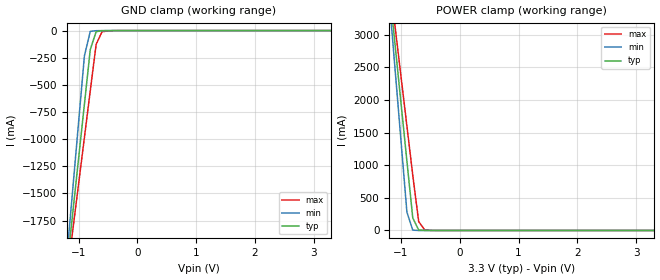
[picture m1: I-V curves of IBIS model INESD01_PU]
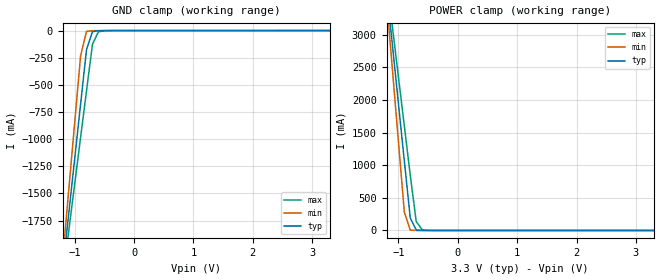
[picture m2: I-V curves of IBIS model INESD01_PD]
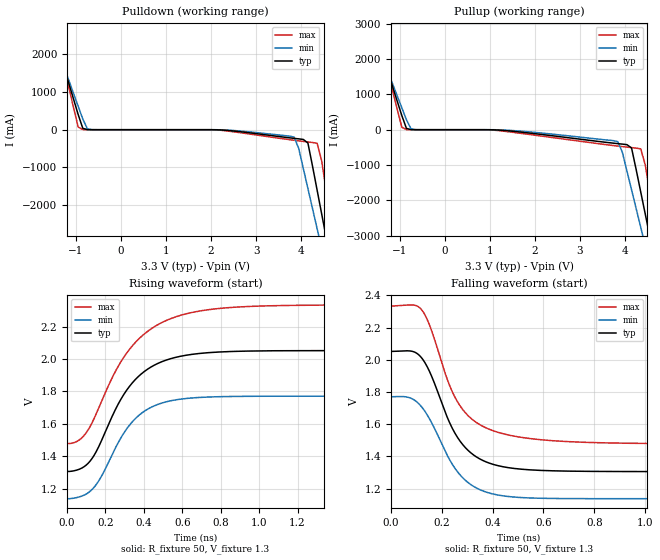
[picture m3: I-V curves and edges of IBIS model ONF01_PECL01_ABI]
|   This file is an IBIS representation of the   |
|   Integrated Devices Technology, Inc.   |
|   ICS84321   |
|   XTAL to 3.3V Differential LVPECL Frequency Synthesizer   |
[IBIS Ver]   4.1
[File name]   84321_3v3.ibs
[File Rev]   1.0
[Date]   31 Dec 2008 | Last modified
|   15 Apr 2003 | Generated
[Source]   Originated at Integrated Devices Technology, Inc.
[Disclaimer]
IDT hereby grants the user of this IBIS model a non-exclusive,
nontransferable license to use this IBIS model under the following terms.
Before using this IBIS model, the user should read this license.
If the user does not accept these terms,  the IBIS model should be
returned to IDT within 30 days.
   The user is granted this license only to use the IBIS model and
is not granted rights to sell, load, rent, lease or license the IBIS
model in whole or in part, or in modified form to anyone other than
user. User may modify the IBIS model to suit its specific
applications but rights to derivative works and such modifications
shall belong to IDT.
   This IBIS model is provided on an "AS IS" basis and IDT makes
absolutely no warranty with respect to the information contained
herein. IDT DISCLAIMS AND CUSTOMER WAIVES ALL WARRANTIES, EXPRESS
OR IMPLIED, INCLUDING WARRANTIES OF MERCHANTABILITY OR FITNESS FOR
A PARTICULAR PURPOSE. The entire risk as to quality and performance
is with the Customer. ACCORDINGLY, IN NO EVENT SHALL THE COMPANY BE
LIABLE FOR ANY DAMAGES, WHETHER IN CONTRACT OR TORT,INCLUDING ANY
LOST PROFITS OR OTHER INCIDENTAL, CONSEQUENTIAL, EXEMPLARY, OR
PUNITIVE DAMAGES ARISING OUT OF THE USE OR APPLICATION OF THE IBIS
model provided in this package. Further, IDT reserves the right to
make changes without notice to any product herein to improve
reliability, function, or design. IDT does not convey any license
under patent rights or any other intellectual property rights,
including those of third parties.
   IDT is not obligated to provide maintenance or support
for the licensed IBIS model.
[Copyright]   Copyright 2003 by Integrated Devices Technology, Inc.
[Component]   ICS84321
[Manufacturer] Integrated Devices Technology, Inc.
[Package]
|LQFP32
|lead+wire  typ   min   max
R_pkg   220.4m   212.5m   238m
L_pkg   1.841n   1.708n   1.974n
C_pkg   0.316p   0.2907p   0.33p
[Pin]   signal_name   model_name   R_pin   L_pin   C_pin
1   M5   INESD01_PU   238m   1.974n   0.330p
2   M6   INESD01_PD   225m   1.841n   0.311p
3   M7   INESD01_PD   218m   1.7745n   0.301p
4   M8   INESD01_PU   213m   1.708n   0.291p
5   NO   INESD01_PU   213m   1.708n   0.291p
6   N1   INESD01_PU   218m   1.7745n   0.301p
7   NC   NC   225m   1.841n   0.311p
8   VEE   GND   238m   1.974n   0.330p
9   TEST   NC   238m   1.974n   0.330p
10   VCC   POWER   225m   1.841n   0.311p
11   FOUT1   ONF01_PECL01_ABI   218m   1.7745n   0.301p
12   nFOUT1   ONF01_PECL01_ABI   213m   1.708n   0.291p
13   VCCO   POWER   213m   1.708n   0.291p
14   FOUT0   ONF01_PECL01_ABI   218m   1.7745n   0.301p
15   nFOUT0   ONF01_PECL01_ABI   225m   1.841n   0.311p
16   VEE   GND   238m   1.974n   0.330p
17   MR   INESD01_PD   238m   1.974n   0.330p
18   S_CLOCK   INESD01_PD   225m   1.841n   0.311p
19   S_DATA   INESD01_PD   218m   1.7745n   0.301p
20   S_LOAD   INESD01_PD   213m   1.708n   0.291p
21   VCCA   POWER   213m   1.708n   0.291p
22   XTAL_SEL   INESD01_PU   218m   1.7745n   0.301p
23   TEST_CLK   INESD01_PD   225m   1.841n   0.311p
24   XTAL_OUT   NC   238m   1.974n   0.330p
25   XTAL_IN   NC   238m   1.974n   0.330p
26   nP_LOAD   INESD01_PD   225m   1.841n   0.311p
27   VCO_SEL   INESD01_PU   218m   1.7745n   0.301p
28   M0   INESD01_PD   213m   1.708n   0.291p
29   M1   INESD01_PD   213m   1.708n   0.291p
30   M2   INESD01_PD   218m   1.7745n   0.301p
31   M3   INESD01_PD   225m   1.841n   0.311p
32   M4   INESD01_PD   238m   1.974n   0.330p
[Diff Pin]  inv_pin  vdiff tdelay_typ tdelay_min  tdelay_max
11   12   NA   0  0  0
14   15   NA   0  0  0
| Models and submodels in the file (3): INESD01_PU (Input), INESD01_PD (Input), ONF01_PECL01_ABI (Output_ECL)
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[Model]   INESD01_PU
Model_type   Input
Polarity   Non-Inverting
Vinl = 0.8V
Vinh = 2.0V
|   typ   min   max
C_comp   2pF   1.5pF   2.5pF
|   typ   min   max
[Voltage range]  3.3V   3.15V   3.45V
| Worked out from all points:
|   GND clamp passes 1 mA (typ) near -0.55 V on its own axis
|   POWER clamp passes 1 mA (typ) near -0.61 V on its own axis
[GND_clamp]
|Voltage   I(typ)   I(min)   I(max)
-3.3V     -12.83A    -15.14A    -11.37A
-1.2V     -2.195A    -2.092A    -2.281A
-1.1V     -1.689A    -1.472A    -1.849A
-900mV    -678.5mA   -232.7mA   -984.8mA
-800mV    -174mA     -7.237mA   -553.3mA
-700mV    -9.767mA   -1.114mA   -126.1mA
-600mV    -1.7mA     -240.1uA   -11.15mA
-300mV    -81.66uA   -67.79uA   -163.4uA
3.3V      1.866nA    1.113pA    239.1nA
[POWER_clamp]
|Voltage   I(typ)   I(min)   I(max)
-3.3V     22.38A     26.45A     19.82A
-1.2V     3.723A     3.545A     3.874A
-1.1V     2.836A     2.457A     3.116A
-1V       1.949A     1.369A     2.358A
-900mV    1.063A     281mA      1.601A
-800mV    191.5mA    5.012mA    843.9mA
-700mV    8.032mA    142.2uA    138.3mA
-600mV    607uA      17.63uA    10.62mA
-400mV    16.32uA    7.545uA    335.9uA
3.3V      -71.13uA   -62.11uA   -78.26uA
[Model]   INESD01_PD
Model_type   Input
Polarity   Non-Inverting
Vinl = 0.80V
Vinh = 2.0V
|   typ   min   max
C_comp   2pF   1.5pF   2.5pF
|   typ   min   max
[Voltage range]  3.3V   3.15V   3.45V
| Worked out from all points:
|   GND clamp passes 1 mA (typ) near -0.55 V on its own axis
|   POWER clamp passes 1 mA (typ) near -0.60 V on its own axis
[GND_clamp]
|Voltage I(typ)   I(min)   I(max)
-3.3V     -12.83A    -15.14A    -11.37A
-1.2V     -2.195A    -2.092A    -2.281A
-1.1V     -1.689A    -1.472A    -1.849A
-900mV    -678.5mA   -232.6mA   -984.8mA
-800mV    -173.9mA   -7.175mA   -553.2mA
-700mV    -9.696mA   -1.052mA   -126mA
-600mV    -1.629mA   -178uA     -11.07mA
-300mV    -10.53uA   -5.678uA   -86.08uA
3.3V      71.13uA    62.11uA    77.58uA
[POWER_clamp]
|Voltage   I(typ)   I(min)   I(max)
-3.3V     22.38A     26.45A     19.82A
-1.2V     3.723A     3.545A     3.874A
-1.1V     2.836A     2.457A     3.116A
-1V       1.949A     1.369A     2.358A
-900mV    1.063A     281.1mA    1.601A
-800mV    191.6mA    5.074mA    844mA
-700mV    8.104mA    204.3uA    138.4mA
-600mV    678.1uA    79.74uA    10.7mA
-400mV    87.44uA    69.65uA    413.2uA
3.3V      -3.041nA   -425fA     -919.9nA
[Model]   ONF01_PECL01_ABI
Model_type  Output_ECL
Polarity   Non-Inverting
Vmeas = 1.63
Rref = 50
Cref = 0
Vref = 1.3
|Variable  typ   min   max
C_comp   2p   1.5p   2.5p
[Voltage Range]   3.3   3.135   3.465
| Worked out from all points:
|   rising waveform, R_fixture 50, V_fixture 1.3: 20-80 % time 218ps typ, 193ps min, 263ps max; typ from 1.31 V to 2.05 V
|   falling waveform, R_fixture 50, V_fixture 1.3: 20-80 % time 134ps typ, 136ps min, 142ps max; typ from 2.05 V to 1.31 V
| Open source, no load
|  Voltage   I(typ)   I(min)   I(max)
[Pulldown]
-3.3V     9.786A     8.425A     12.06A
-1.667V   3.247A     2.986A     3.704A
-1.463V   2.432A     2.308A     2.661A
-952.6mV  398mA      618.5mA    68.87mA
-850.5mV  36.63mA    281.6mA    4.032mA
3.844V    -229.1mA   -195.7mA   -279.4mA
4.151V    -352.7mA   -1.559A    -324.9mA
4.355V    -1.599A    -2.62A     -360.9mA
4.559V    -2.871A    -3.681A    -1.635A
4.661V    -3.508A    -4.211A    -2.446A
4.763V    -4.144A    -4.742A    -3.257A
6.6V      -15.69A    -14.35A    -17.99A
[Pullup]
-3.3V     9.786A     8.425A     12.06A
-1.565V   2.839A     2.647A     3.182A
-952.6mV  398mA      618.5mA    68.87mA
-850.5mV  36.63mA    281.6mA    4.032mA
-646.4mV  229.3uA    964.8uA    177.5uA
3.844V    -394.4mA   -337mA     -463.1mA
4.151V    -517.8mA   -1.701A    -507.4mA
4.355V    -1.764A    -2.763A    -542.7mA
4.559V    -3.036A    -3.825A    -1.816A
4.661V    -3.672A    -4.355A    -2.626A
4.763V    -4.308A    -4.886A    -3.437A
6.6V      -15.79A    -14.46A    -18.06A
[Ramp]
|   typ   min   max
dV/dt_r   0.596/0.354n   0.506/0.311n   0.684/0.427n
dV/dt_f   0.599/0.219n   0.507/0.219n   0.690/0.252n
R_load =   50.0000
[Rising Waveform]
R_fixture = 50
V_fixture = 1.3   | VCC_typ - 2V
V_fixture_max = 1.465   | VCC_max - 2V
V_fixture_min = 1.135   | VCC_min - 2V
C_fixture = 0.0p
| Time   typ   min   max
0s        1.306V     1.138V     1.478V
67.2ps    1.321V     1.15V      1.503V
126ps     1.379V     1.19V      1.597V
176.4ps   1.489V     1.271V     1.731V
247.8ps   1.679V     1.442V     1.915V
338.1ps   1.85V      1.61V      2.079V
430.5ps   1.946V     1.698V     2.18V
554.4ps   2.007V     1.745V     2.255V
936.6ps   2.049V     1.77V      2.324V
1.999ns   2.052V     1.771V     2.333V
[Falling Waveform]
R_fixture = 50
V_fixture = 1.3   | VCC_typ - 2V
V_fixture_max = 1.465   | VCC_max - 2V
V_fixture_min = 1.135   | VCC_min - 2V
C_fixture = 0.0p
| Time   typ   min   max
0s        2.052V     1.771V     2.334V
73.5ps    2.055V     1.765V     2.34V
119.7ps   2.015V     1.711V     2.314V
151.2ps   1.932V     1.637V     2.221V
224.7ps   1.633V     1.399V     1.868V
268.8ps   1.503V     1.293V     1.723V
336ps     1.398V     1.205V     1.611V
434.7ps   1.338V     1.157V     1.544V
806.4ps   1.307V     1.138V     1.486V
1.999ns   1.306V     1.138V     1.478V
